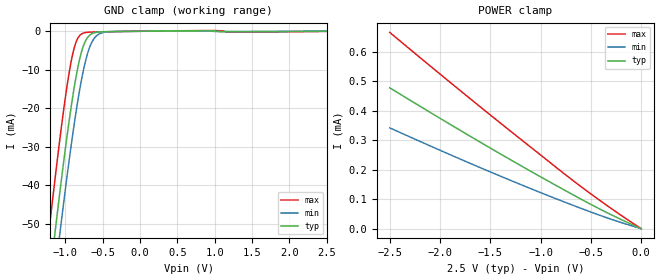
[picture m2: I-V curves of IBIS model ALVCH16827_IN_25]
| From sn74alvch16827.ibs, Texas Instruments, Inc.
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[Model]   ALVCH16827_IN_25
Model_type  Input
Vinl=0.7
Vinh=1.7
| variable   typ   min   max
C_comp   1.95pF   1.63pF   2.21pF
[Temperature Range]   40   100   -40
| Ambient temperature   25   85   -40
[Voltage range]   2.5   2.3   2.7
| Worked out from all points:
|   GND clamp passes 1 mA (typ) near -0.67 V on its own axis
[GND Clamp]
| ALVCH16827_IN_25
|   Voltage   I(typ)   I(min)   I(max)
-2.5V     -300.6mA   -309.9mA   -289.2mA
-1.22V    -66.2mA    -76.97mA   -52.37mA
-1.15V    -54.46mA   -65.25mA   -40.58mA
-1.125V   -50.35mA   -61.13mA   -36.48mA
-1.07V    -41.51mA   -52.24mA   -27.74mA
-980mV    -27.85mA   -38.29mA   -14.78mA
-910mV    -18.28mA   -28.19mA   -6.818mA
-845mV    -10.77mA   -19.67mA   -2.339mA
-770mV    -4.568mA   -11.37mA   -584.1uA
-645mV    -658.2uA   -2.897mA   -211.8uA
-485mV    -121.3uA   -296.5uA   -146.6uA
2.5V      1.114nA    20.81uA    -42.68uA
[POWER Clamp]
| ALVCH16827_IN_25
|   Voltage   I(typ)   I(min)   I(max)
-2.5V     477.5uA    341.7uA    665.3uA
-1.605V   294.2uA    207.5uA    414.3uA
-775mV    133uA      91.91uA    188.8uA
-380mV    61.1uA     41.52uA    88.18uA
-31.15fV  1.114nA    59.61nA    7.152pA
